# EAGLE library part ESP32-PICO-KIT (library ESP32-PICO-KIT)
Esp32 Wifi Bluetooth Eval Board
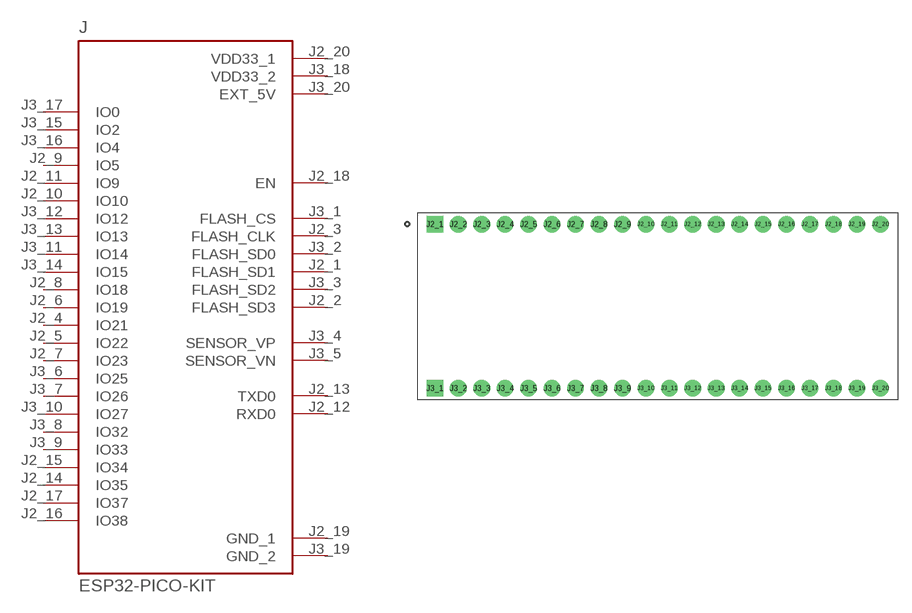
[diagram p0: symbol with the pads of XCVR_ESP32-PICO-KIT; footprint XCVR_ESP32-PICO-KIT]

Designator prefix J

## ESP32-PICO-KIT (Availability: Unavailable; Description: - Transceiver; 802.11 b/g/n _Wi-Fi, WiFi, WLAN_, Bluetooth® Smart Ready 4.x Dual Mode For Use With ESP32-PICO-D4; MF: Espressif Systems; MP: ESP32-PICO-KIT; Package: None; Price: None)  [XCVR_ESP32-PICO-KIT]
J2_1  FLASH_SD1
J2_2  FLASH_SD3
J2_3  FLASH_CLK
J2_4  IO21
J2_5  IO22
J2_6  IO19
J2_7  IO23
J2_8  IO18
J2_9  IO5
J2_10  IO10
J2_11  IO9
J2_12  RXD0
J2_13  TXD0
J2_14  IO35  in
J2_15  IO34  in
J2_16  IO38  in
J2_17  IO37  in
J2_18  EN  in
J2_19  GND_1  pwr
J2_20  VDD33_1  pwr
J3_1  FLASH_CS
J3_2  FLASH_SD0
J3_3  FLASH_SD2
J3_4  SENSOR_VP  in
J3_5  SENSOR_VN  in
J3_6  IO25
J3_7  IO26
J3_8  IO32
J3_9  IO33
J3_10  IO27
J3_11  IO14
J3_12  IO12
J3_13  IO13
J3_14  IO15
J3_15  IO2
J3_16  IO4
J3_17  IO0
J3_18  VDD33_2  pwr
J3_19  GND_2  pwr
J3_20  EXT_5V  pwr

## Footprint XCVR_ESP32-PICO-KIT (pad centres in mm)
drill 1.2 square: J2_1 -24.13,8.89; J3_1 -24.13,-8.89
drill 1.2: J2_2 -21.59,8.89; J2_3 -19.05,8.89; J2_4 -16.51,8.89; J2_5 -13.97,8.89; J2_6 -11.43,8.89; J2_7 -8.89,8.89; J2_8 -6.35,8.89; J2_9 -3.81,8.89; J2_10 -1.27,8.89; J2_11 1.27,8.89; J2_12 3.81,8.89; J2_13 6.35,8.89; J2_14 8.89,8.89; J2_15 11.43,8.89; J2_16 13.97,8.89; J2_17 16.51,8.89; J2_18 19.05,8.89; J2_19 21.59,8.89; J2_20 24.13,8.89; J3_2 -21.59,-8.89; J3_3 -19.05,-8.89; J3_4 -16.51,-8.89; J3_5 -13.97,-8.89; J3_6 -11.43,-8.89; J3_7 -8.89,-8.89; J3_8 -6.35,-8.89; J3_9 -3.81,-8.89; J3_10 -1.27,-8.89; J3_11 1.27,-8.89; J3_12 3.81,-8.89; J3_13 6.35,-8.89; J3_14 8.89,-8.89; J3_15 11.43,-8.89; J3_16 13.97,-8.89; J3_17 16.51,-8.89; J3_18 19.05,-8.89; J3_19 21.59,-8.89; J3_20 24.13,-8.89

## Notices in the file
This work is licensed under a Creative Commons Attribution-ShareAlike 4.0 International License (CC BY-SA) with Design Exception 1.0
